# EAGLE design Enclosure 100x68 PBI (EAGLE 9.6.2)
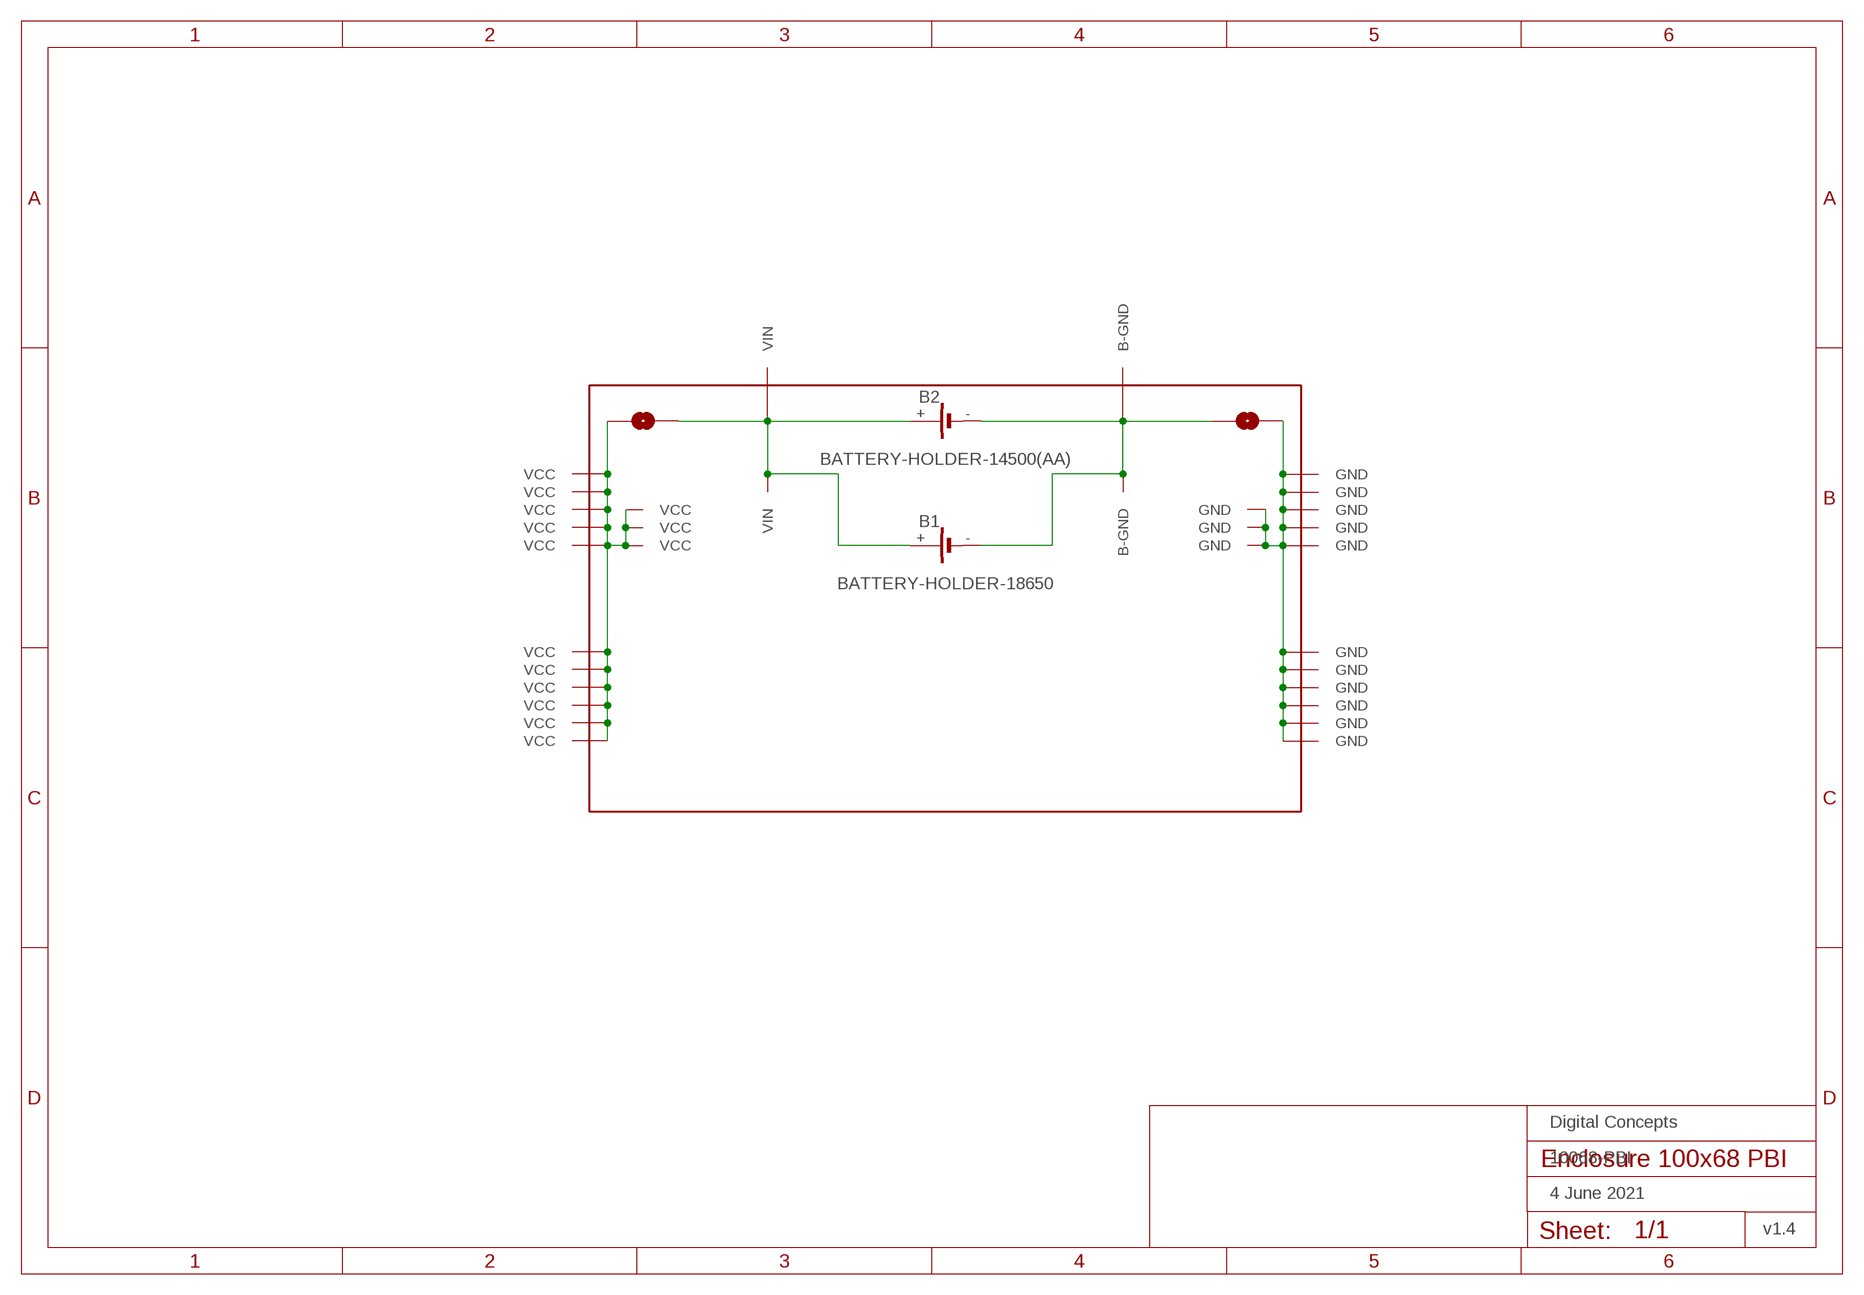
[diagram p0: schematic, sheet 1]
FRAME1 (FRAME-A4L-LOC): DATE: 4 June 2021; OWNER: Digital Concepts; TITLE: 10068-PBI; VERSION: v1.4

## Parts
B1  BATTERY-HOLDER-18650  [BATTERY-18650]
B2  BATTERY-HOLDER-14500(AA)  [BATTERY-14500]
P1  PROTO-34X22-BAT-SJ-MK2  [PROTO-34X22-BAT-SJ-MK2]

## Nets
GND: P1.GND P1.P33-13(GND) P1.P33-14(GND) P1.P33-15(GND) P1.P34-05(GND) P1.P34-06(GND) P1.P34-07(GND) P1.P34-08(GND) P1.P34-09(GND) P1.P34-10(GND) P1.P34-13(GND) P1.P34-14(GND) P1.P34-15(GND) P1.P34-16(GND) P1.P34-17(GND)
N$3: B1.+ B2.+ P1.P02-17(VIN) P1.P05-19(VIN) P1.VIN
N$4: B1.- B2.- P1.B-GND P1.P30-19(B-GND) P1.P33-17(B-GND)
VCC: P1.P01-05(VCC) P1.P01-06(VCC) P1.P01-07(VCC) P1.P01-08(VCC) P1.P01-09(VCC) P1.P01-10(VCC) P1.P01-13(VCC) P1.P01-14(VCC) P1.P01-15(VCC) P1.P01-16(VCC) P1.P01-17(VCC) P1.P02-13(VCC) P1.P02-14(VCC) P1.P02-15(VCC) P1.VCC

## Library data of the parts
B1 = digitalconcepts:BATTERY-HOLDER-18650: 18650 Battery Holder
B2 = digitalconcepts:BATTERY-HOLDER-14500(AA): 14500 (AA) battery holder
P1 = digitalconcepts:PROTO-34X22-BAT-SJ-MK2: 34 x 22 Prototyping board, with spaces for battery connection (GND + Vcc plane) to fit a 100 x 68 enclosure

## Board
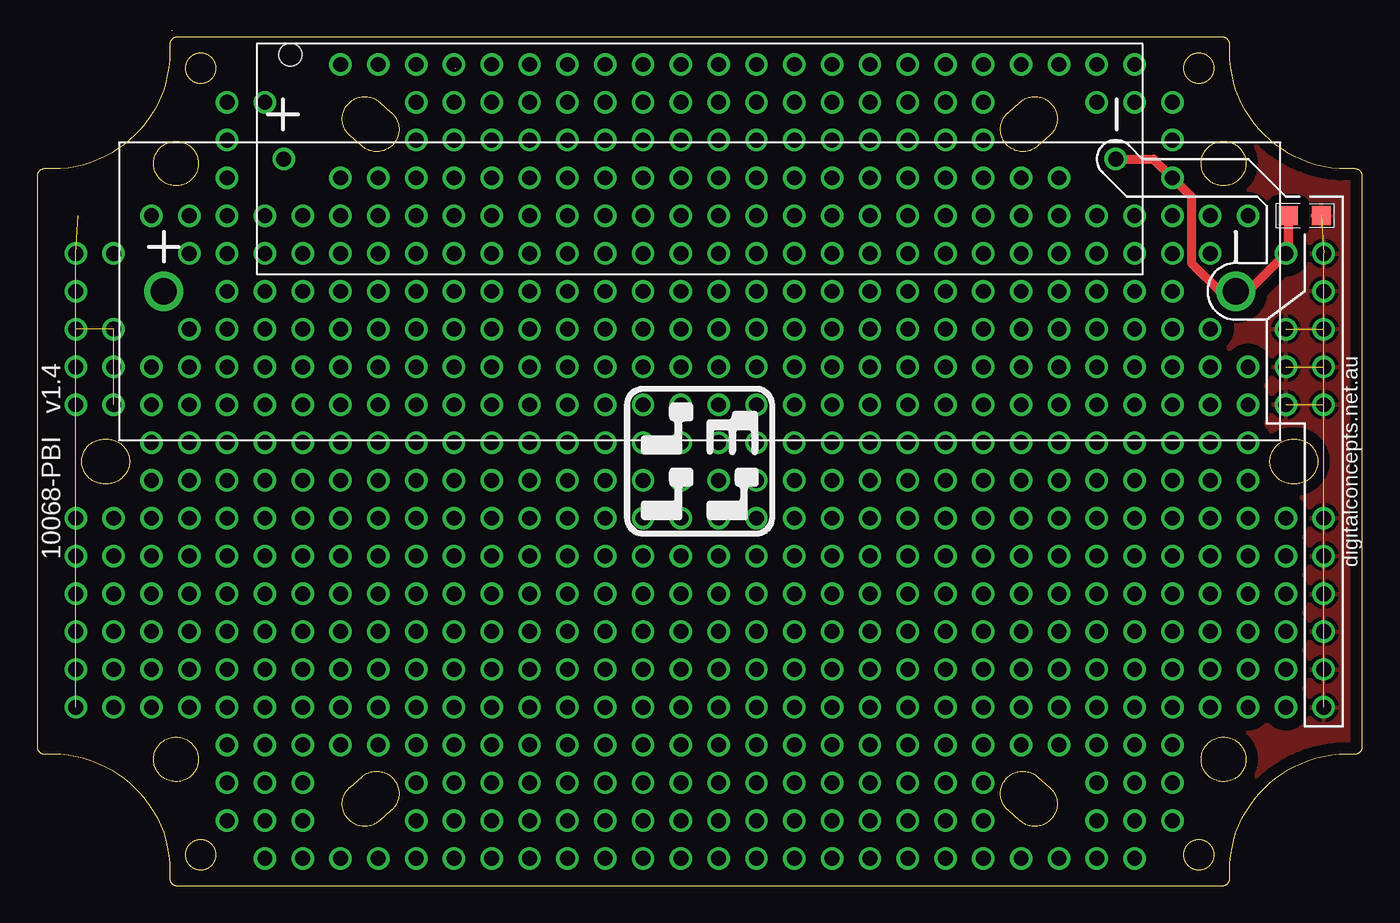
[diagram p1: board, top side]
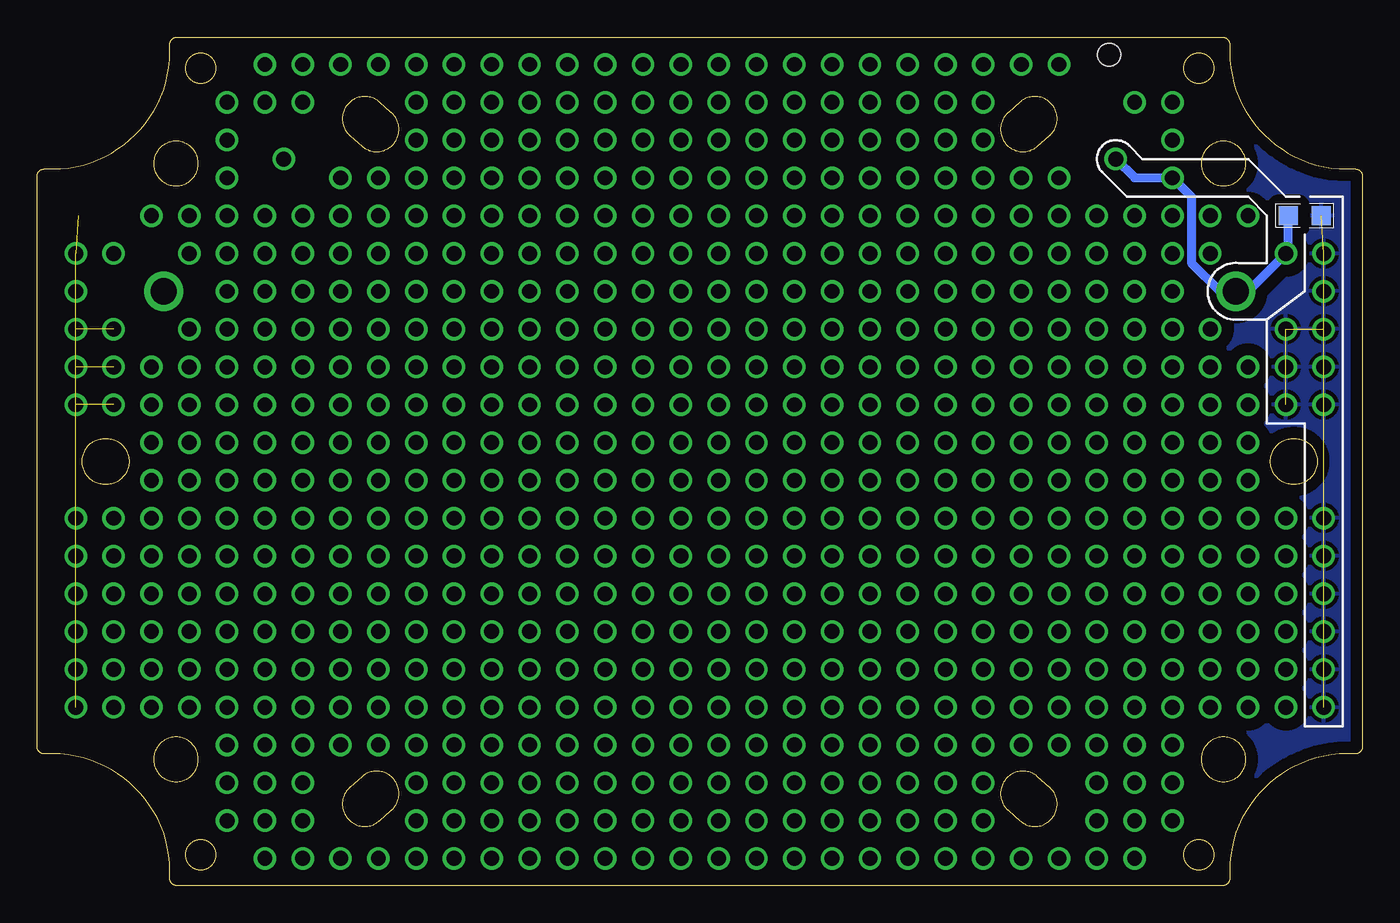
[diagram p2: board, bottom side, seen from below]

Size 89 x 57 mm. Coordinates in mm from the lower left corner, seen from the top.
Outline: 1238 segments
Outline: circle at 10.97,54.92 radius 1.02
Outline: circle at 78.03,54.92 radius 1.02
Outline: circle at 78.03,2.08 radius 1.02
Outline: circle at 10.97,2.08 radius 1.02
Copper layers (1*16): Top 0.035mm / dielectric 1.5mm / Bottom 0.035mm
Design rules "default *": minimum track width 6mil, minimum drill 0.35mm, track to track 6mil, track to pad 6mil, pad to pad 6mil, via to via 6mil, smd to smd 6mil, copper to edge 6mil, drill to drill 6mil, minimum pad ring 10mil, minimum via ring 8mil, stop-mask expansion 4mil, vias tented up to drill 0mil, thermal gap 10mil

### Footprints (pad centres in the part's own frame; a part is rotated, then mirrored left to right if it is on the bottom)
BATTERY-18650 = drill 1.75: + -36,0; - 36,0
BATTERY-14500 = drill 1: + -27.94,0; - 27.94,0 | hole 1.524: -27.5,7
PROTO-34X22-BAT-SJ-MK2 = smd 1.27 x 1.27: B-GND 39.534,16.51; GND 41.746,16.51 | drill 1: P01-05 -41.91,-16.51; P01-06 -41.91,-13.97; P01-07 -41.91,-11.43; P01-08 -41.91,-8.89; P01-09 -41.91,-6.35; P01-10 -41.91,-3.81; P01-13 -41.91,3.81; P01-14 -41.91,6.35; P01-15 -41.91,8.89; P01-16 -41.91,11.43; P01-17 -41.91,13.97; P02-05 -39.37,-16.51; P02-06 -39.37,-13.97; P02-07 -39.37,-11.43; P02-08 -39.37,-8.89; P02-09 -39.37,-6.35; P02-10 -39.37,-3.81; P02-13 -39.37,3.81; P02-14 -39.37,6.35; P02-15 -39.37,8.89; P02-17 -39.37,13.97; P03-05 -36.83,-16.51; P03-06 -36.83,-13.97; P03-07 -36.83,-11.43; P03-08 -36.83,-8.89; P03-09 -36.83,-6.35; P03-10 -36.83,-3.81; P03-11 -36.83,-1.27; P03-12 -36.83,1.27; P03-13 -36.83,3.81; P03-14 -36.83,6.35; P03-18 -36.83,16.51; P04-05 -34.29,-16.51; P04-06 -34.29,-13.97; P04-07 -34.29,-11.43; P04-08 -34.29,-8.89; P04-09 -34.29,-6.35; P04-10 -34.29,-3.81; P04-11 -34.29,-1.27; P04-12 -34.29,1.27; P04-13 -34.29,3.81; P04-14 -34.29,6.35; P04-15 -34.29,8.89; P04-17 -34.29,13.97; P04-18 -34.29,16.51; P05-02 -31.75,-24.13; P05-03 -31.75,-21.59; P05-04 -31.75,-19.05; P05-05 -31.75,-16.51; P05-06 -31.75,-13.97; P05-07 -31.75,-11.43; P05-08 -31.75,-8.89; P05-09 -31.75,-6.35; P05-10 -31.75,-3.81; P05-11 -31.75,-1.27; P05-12 -31.75,1.27; P05-13 -31.75,3.81; P05-14 -31.75,6.35; P05-15 -31.75,8.89; P05-16 -31.75,11.43; P05-17 -31.75,13.97; P05-18 -31.75,16.51; P05-19 -31.75,19.05; P05-20 -31.75,21.59; P05-21 -31.75,24.13; P06-01 -29.21,-26.67; P06-02 -29.21,-24.13; P06-03 -29.21,-21.59; P06-04 -29.21,-19.05; P06-05 -29.21,-16.51; P06-06 -29.21,-13.97; P06-07 -29.21,-11.43; P06-08 -29.21,-8.89; P06-09 -29.21,-6.35; P06-10 -29.21,-3.81; P06-11 -29.21,-1.27; P06-12 -29.21,1.27; P06-13 -29.21,3.81; P06-14 -29.21,6.35; P06-15 -29.21,8.89; P06-16 -29.21,11.43; P06-17 -29.21,13.97; P06-18 -29.21,16.51; P06-21 -29.21,24.13; P07-01 -26.67,-26.67; P07-02 -26.67,-24.13; P07-03 -26.67,-21.59; P07-04 -26.67,-19.05; P07-05 -26.67,-16.51; P07-06 -26.67,-13.97; P07-07 -26.67,-11.43; P07-08 -26.67,-8.89; P07-09 -26.67,-6.35; P07-10 -26.67,-3.81; P07-11 -26.67,-1.27; P07-12 -26.67,1.27; P07-13 -26.67,3.81; P07-14 -26.67,6.35; P07-15 -26.67,8.89; P07-16 -26.67,11.43; P07-17 -26.67,13.97; P07-18 -26.67,16.51; P08-01 -24.13,-26.67; P08-04 -24.13,-19.05; P08-05 -24.13,-16.51; P08-06 -24.13,-13.97; P08-07 -24.13,-11.43; P08-08 -24.13,-8.89; P08-09 -24.13,-6.35; P08-10 -24.13,-3.81; P08-11 -24.13,-1.27; P08-12 -24.13,1.27; P08-13 -24.13,3.81; P08-14 -24.13,6.35; P08-15 -24.13,8.89; P08-16 -24.13,11.43; P08-17 -24.13,13.97; P08-18 -24.13,16.51; P08-19 -24.13,19.05; P08-22 -24.13,26.67; P09-01 -21.59,-26.67; P09-04 -21.59,-19.05; P09-05 -21.59,-16.51; P09-06 -21.59,-13.97; P09-07 -21.59,-11.43; P09-08 -21.59,-8.89; P09-09 -21.59,-6.35; P09-10 -21.59,-3.81; P09-11 -21.59,-1.27; P09-12 -21.59,1.27; P09-13 -21.59,3.81; P09-14 -21.59,6.35; P09-15 -21.59,8.89; P09-16 -21.59,11.43; P09-17 -21.59,13.97; P09-18 -21.59,16.51; P09-19 -21.59,19.05; P09-22 -21.59,26.67; P10-01 -19.05,-26.67; P10-02 -19.05,-24.13; P10-03 -19.05,-21.59; P10-04 -19.05,-19.05; P10-05 -19.05,-16.51; P10-06 -19.05,-13.97; P10-07 -19.05,-11.43; P10-08 -19.05,-8.89; P10-09 -19.05,-6.35; P10-10 -19.05,-3.81; P10-11 -19.05,-1.27; P10-12 -19.05,1.27; P10-13 -19.05,3.81; P10-14 -19.05,6.35; P10-15 -19.05,8.89; P10-16 -19.05,11.43; P10-17 -19.05,13.97; P10-18 -19.05,16.51; P10-19 -19.05,19.05; P10-20 -19.05,21.59; P10-21 -19.05,24.13; P10-22 -19.05,26.67; P11-01 -16.51,-26.67; P11-02 -16.51,-24.13; P11-03 -16.51,-21.59; P11-04 -16.51,-19.05; P11-05 -16.51,-16.51; P11-06 -16.51,-13.97; P11-07 -16.51,-11.43; P11-08 -16.51,-8.89; P11-09 -16.51,-6.35; P11-10 -16.51,-3.81; P11-11 -16.51,-1.27; P11-12 -16.51,1.27; P11-13 -16.51,3.81; P11-14 -16.51,6.35; P11-15 -16.51,8.89; P11-16 -16.51,11.43; P11-17 -16.51,13.97; P11-18 -16.51,16.51; P11-19 -16.51,19.05; P11-20 -16.51,21.59; P11-21 -16.51,24.13; P11-22 -16.51,26.67; P12-01 -13.97,-26.67; P12-02 -13.97,-24.13; P12-03 -13.97,-21.59; P12-04 -13.97,-19.05; P12-05 -13.97,-16.51; P12-06 -13.97,-13.97; P12-07 -13.97,-11.43; P12-08 -13.97,-8.89; P12-09 -13.97,-6.35; P12-10 -13.97,-3.81; P12-11 -13.97,-1.27; P12-12 -13.97,1.27; P12-13 -13.97,3.81; P12-14 -13.97,6.35; P12-15 -13.97,8.89; P12-16 -13.97,11.43; P12-17 -13.97,13.97; P12-18 -13.97,16.51; P12-19 -13.97,19.05; P12-20 -13.97,21.59; P12-21 -13.97,24.13; P12-22 -13.97,26.67; P13-01 -11.43,-26.67; P13-02 -11.43,-24.13; P13-03 -11.43,-21.59; P13-04 -11.43,-19.05; P13-05 -11.43,-16.51; P13-06 -11.43,-13.97; P13-07 -11.43,-11.43; P13-08 -11.43,-8.89; P13-09 -11.43,-6.35; P13-10 -11.43,-3.81; P13-11 -11.43,-1.27; P13-12 -11.43,1.27; P13-13 -11.43,3.81; P13-14 -11.43,6.35; P13-15 -11.43,8.89; P13-16 -11.43,11.43; P13-17 -11.43,13.97; P13-18 -11.43,16.51; P13-19 -11.43,19.05; P13-20 -11.43,21.59; P13-21 -11.43,24.13; P13-22 -11.43,26.67; P14-01 -8.89,-26.67; P14-02 -8.89,-24.13; P14-03 -8.89,-21.59; P14-04 -8.89,-19.05; P14-05 -8.89,-16.51; P14-06 -8.89,-13.97; P14-07 -8.89,-11.43; P14-08 -8.89,-8.89; P14-09 -8.89,-6.35; P14-10 -8.89,-3.81; P14-11 -8.89,-1.27; P14-12 -8.89,1.27; P14-13 -8.89,3.81; P14-14 -8.89,6.35; P14-15 -8.89,8.89; P14-16 -8.89,11.43; P14-17 -8.89,13.97; P14-18 -8.89,16.51; P14-19 -8.89,19.05; P14-20 -8.89,21.59; P14-21 -8.89,24.13; P14-22 -8.89,26.67; P15-01 -6.35,-26.67; P15-02 -6.35,-24.13; P15-03 -6.35,-21.59; P15-04 -6.35,-19.05; P15-05 -6.35,-16.51; P15-06 -6.35,-13.97; P15-07 -6.35,-11.43; P15-08 -6.35,-8.89; P15-09 -6.35,-6.35; P15-10 -6.35,-3.81; P15-11 -6.35,-1.27; P15-12 -6.35,1.27; P15-13 -6.35,3.81; P15-14 -6.35,6.35; P15-15 -6.35,8.89; P15-16 -6.35,11.43; P15-17 -6.35,13.97; P15-18 -6.35,16.51; P15-19 -6.35,19.05; P15-20 -6.35,21.59; P15-21 -6.35,24.13; P15-22 -6.35,26.67; P16-01 -3.81,-26.67; P16-02 -3.81,-24.13; P16-03 -3.81,-21.59; P16-04 -3.81,-19.05; P16-05 -3.81,-16.51; P16-06 -3.81,-13.97; P16-07 -3.81,-11.43; P16-08 -3.81,-8.89; P16-09 -3.81,-6.35; P16-10 -3.81,-3.81; P16-11 -3.81,-1.27; P16-12 -3.81,1.27; P16-13 -3.81,3.81; P16-14 -3.81,6.35; P16-15 -3.81,8.89; P16-16 -3.81,11.43; P16-17 -3.81,13.97; P16-18 -3.81,16.51; P16-19 -3.81,19.05; P16-20 -3.81,21.59; P16-21 -3.81,24.13; P16-22 -3.81,26.67; P17-01 -1.27,-26.67; P17-02 -1.27,-24.13; P17-03 -1.27,-21.59; P17-04 -1.27,-19.05; P17-05 -1.27,-16.51; P17-06 -1.27,-13.97; P17-07 -1.27,-11.43; P17-08 -1.27,-8.89; P17-09 -1.27,-6.35; P17-10 -1.27,-3.81; P17-11 -1.27,-1.27; P17-12 -1.27,1.27; P17-13 -1.27,3.81; P17-14 -1.27,6.35; P17-15 -1.27,8.89; P17-16 -1.27,11.43; P17-17 -1.27,13.97; P17-18 -1.27,16.51; P17-19 -1.27,19.05; P17-20 -1.27,21.59; P17-21 -1.27,24.13; P17-22 -1.27,26.67; P18-01 1.27,-26.67; P18-02 1.27,-24.13; P18-03 1.27,-21.59; P18-04 1.27,-19.05; P18-05 1.27,-16.51; P18-06 1.27,-13.97; P18-07 1.27,-11.43; P18-08 1.27,-8.89; P18-09 1.27,-6.35; P18-10 1.27,-3.81; P18-11 1.27,-1.27; P18-12 1.27,1.27; P18-13 1.27,3.81; P18-14 1.27,6.35; P18-15 1.27,8.89; P18-16 1.27,11.43; P18-17 1.27,13.97; P18-18 1.27,16.51; P18-19 1.27,19.05; P18-20 1.27,21.59; P18-21 1.27,24.13; P18-22 1.27,26.67; P19-01 3.81,-26.67; P19-02 3.81,-24.13; P19-03 3.81,-21.59; P19-04 3.81,-19.05; P19-05 3.81,-16.51; P19-06 3.81,-13.97; P19-07 3.81,-11.43; P19-08 3.81,-8.89; P19-09 3.81,-6.35; P19-10 3.81,-3.81; P19-11 3.81,-1.27; P19-12 3.81,1.27; P19-13 3.81,3.81; P19-14 3.81,6.35; P19-15 3.81,8.89; P19-16 3.81,11.43; P19-17 3.81,13.97; P19-18 3.81,16.51; P19-19 3.81,19.05; P19-20 3.81,21.59; P19-21 3.81,24.13; P19-22 3.81,26.67; P20-01 6.35,-26.67; P20-02 6.35,-24.13; P20-03 6.35,-21.59; P20-04 6.35,-19.05; P20-05 6.35,-16.51; P20-06 6.35,-13.97; P20-07 6.35,-11.43; P20-08 6.35,-8.89; P20-09 6.35,-6.35; P20-10 6.35,-3.81; P20-11 6.35,-1.27; P20-12 6.35,1.27; P20-13 6.35,3.81; P20-14 6.35,6.35; P20-15 6.35,8.89; P20-16 6.35,11.43; P20-17 6.35,13.97; P20-18 6.35,16.51; P20-19 6.35,19.05; P20-20 6.35,21.59; P20-21 6.35,24.13; P20-22 6.35,26.67; P21-01 8.89,-26.67; P21-02 8.89,-24.13; P21-03 8.89,-21.59; P21-04 8.89,-19.05; P21-05 8.89,-16.51; P21-06 8.89,-13.97; P21-07 8.89,-11.43; P21-08 8.89,-8.89; P21-09 8.89,-6.35; P21-10 8.89,-3.81; P21-11 8.89,-1.27; P21-12 8.89,1.27; P21-13 8.89,3.81; P21-14 8.89,6.35; P21-15 8.89,8.89; P21-16 8.89,11.43; P21-17 8.89,13.97; P21-18 8.89,16.51; P21-19 8.89,19.05; P21-20 8.89,21.59; P21-21 8.89,24.13; P21-22 8.89,26.67; P22-01 11.43,-26.67; P22-02 11.43,-24.13; P22-03 11.43,-21.59; P22-04 11.43,-19.05; P22-05 11.43,-16.51; P22-06 11.43,-13.97; P22-07 11.43,-11.43; P22-08 11.43,-8.89; P22-09 11.43,-6.35; P22-10 11.43,-3.81; P22-11 11.43,-1.27; P22-12 11.43,1.27; P22-13 11.43,3.81; P22-14 11.43,6.35; P22-15 11.43,8.89; P22-16 11.43,11.43; P22-17 11.43,13.97; P22-18 11.43,16.51; P22-19 11.43,19.05; P22-20 11.43,21.59; P22-21 11.43,24.13; P22-22 11.43,26.67; P23-01 13.97,-26.67; P23-02 13.97,-24.13; P23-03 13.97,-21.59; P23-04 13.97,-19.05; P23-05 13.97,-16.51; P23-06 13.97,-13.97; P23-07 13.97,-11.43; P23-08 13.97,-8.89; P23-09 13.97,-6.35; P23-10 13.97,-3.81; P23-11 13.97,-1.27; P23-12 13.97,1.27; P23-13 13.97,3.81; P23-14 13.97,6.35; P23-15 13.97,8.89; P23-16 13.97,11.43; P23-17 13.97,13.97; P23-18 13.97,16.51; P23-19 13.97,19.05; P23-20 13.97,21.59; P23-21 13.97,24.13; P23-22 13.97,26.67; P24-01 16.51,-26.67; P24-02 16.51,-24.13; P24-03 16.51,-21.59; P24-04 16.51,-19.05; P24-05 16.51,-16.51; P24-06 16.51,-13.97; P24-07 16.51,-11.43; P24-08 16.51,-8.89; P24-09 16.51,-6.35; P24-10 16.51,-3.81; P24-11 16.51,-1.27; P24-12 16.51,1.27; P24-13 16.51,3.81; P24-14 16.51,6.35; P24-15 16.51,8.89; P24-16 16.51,11.43; P24-17 16.51,13.97; P24-18 16.51,16.51; P24-19 16.51,19.05; P24-20 16.51,21.59; P24-21 16.51,24.13; P24-22 16.51,26.67; P25-01 19.05,-26.67; P25-02 19.05,-24.13; P25-03 19.05,-21.59; P25-04 19.05,-19.05; P25-05 19.05,-16.51; P25-06 19.05,-13.97; P25-07 19.05,-11.43; P25-08 19.05,-8.89; P25-09 19.05,-6.35; P25-10 19.05,-3.81; P25-11 19.05,-1.27; P25-12 19.05,1.27; P25-13 19.05,3.81; P25-14 19.05,6.35; P25-15 19.05,8.89; P25-16 19.05,11.43; P25-17 19.05,13.97; P25-18 19.05,16.51; P25-19 19.05,19.05; P25-20 19.05,21.59; P25-21 19.05,24.13; P25-22 19.05,26.67; P26-01 21.59,-26.67; P26-04 21.59,-19.05; P26-05 21.59,-16.51; P26-06 21.59,-13.97; P26-07 21.59,-11.43; P26-08 21.59,-8.89; P26-09 21.59,-6.35; P26-10 21.59,-3.81; P26-11 21.59,-1.27; P26-12 21.59,1.27; P26-13 21.59,3.81; P26-14 21.59,6.35; P26-15 21.59,8.89; P26-16 21.59,11.43; P26-17 21.59,13.97; P26-18 21.59,16.51; P26-19 21.59,19.05; P26-22 21.59,26.67; P27-01 24.13,-26.67; P27-04 24.13,-19.05; P27-05 24.13,-16.51; P27-06 24.13,-13.97; P27-07 24.13,-11.43; P27-08 24.13,-8.89; P27-09 24.13,-6.35; P27-10 24.13,-3.81; P27-11 24.13,-1.27; P27-12 24.13,1.27; P27-13 24.13,3.81; P27-14 24.13,6.35; P27-15 24.13,8.89; P27-16 24.13,11.43; P27-17 24.13,13.97; P27-18 24.13,16.51; P27-19 24.13,19.05; P27-22 24.13,26.67; P28-01 26.67,-26.67; P28-02 26.67,-24.13; P28-03 26.67,-21.59; P28-04 26.67,-19.05; P28-05 26.67,-16.51; P28-06 26.67,-13.97; P28-07 26.67,-11.43; P28-08 26.67,-8.89; P28-09 26.67,-6.35; P28-10 26.67,-3.81; P28-11 26.67,-1.27; P28-12 26.67,1.27; P28-13 26.67,3.81; P28-14 26.67,6.35; P28-15 26.67,8.89; P28-16 26.67,11.43; P28-17 26.67,13.97; P28-18 26.67,16.51; P28-21 26.67,24.13; P28-22 26.67,26.67; P29-01 29.21,-26.67; P29-02 29.21,-24.13; P29-03 29.21,-21.59; P29-04 29.21,-19.05; P29-05 29.21,-16.51; P29-06 29.21,-13.97; P29-07 29.21,-11.43; P29-08 29.21,-8.89; P29-09 29.21,-6.35; P29-10 29.21,-3.81; P29-11 29.21,-1.27; P29-12 29.21,1.27; P29-13 29.21,3.81; P29-14 29.21,6.35; P29-15 29.21,8.89; P29-16 29.21,11.43; P29-17 29.21,13.97; P29-18 29.21,16.51; P29-21 29.21,24.13; P29-22 29.21,26.67; P30-02 31.75,-24.13; P30-03 31.75,-21.59; P30-04 31.75,-19.05; P30-05 31.75,-16.51; P30-06 31.75,-13.97; P30-07 31.75,-11.43; P30-08 31.75,-8.89; P30-09 31.75,-6.35; P30-10 31.75,-3.81; P30-11 31.75,-1.27; P30-12 31.75,1.27; P30-13 31.75,3.81; P30-14 31.75,6.35; P30-15 31.75,8.89; P30-16 31.75,11.43; P30-17 31.75,13.97; P30-18 31.75,16.51; P30-19 31.75,19.05; P30-20 31.75,21.59; P30-21 31.75,24.13; P31-05 34.29,-16.51; P31-06 34.29,-13.97; P31-07 34.29,-11.43; P31-08 34.29,-8.89; P31-09 34.29,-6.35; P31-10 34.29,-3.81; P31-11 34.29,-1.27; P31-12 34.29,1.27; P31-13 34.29,3.81; P31-14 34.29,6.35; P31-15 34.29,8.89; P31-17 34.29,13.97; P31-18 34.29,16.51; P32-05 36.83,-16.51; P32-06 36.83,-13.97; P32-07 36.83,-11.43; P32-08 36.83,-8.89; P32-09 36.83,-6.35; P32-10 36.83,-3.81; P32-11 36.83,-1.27; P32-12 36.83,1.27; P32-13 36.83,3.81; P32-14 36.83,6.35; P32-18 36.83,16.51; P33-05 39.37,-16.51; P33-06 39.37,-13.97; P33-07 39.37,-11.43; P33-08 39.37,-8.89; P33-09 39.37,-6.35; P33-10 39.37,-3.81; P33-13 39.37,3.81; P33-14 39.37,6.35; P33-15 39.37,8.89; P33-17 39.37,13.97; P34-05 41.91,-16.51; P34-06 41.91,-13.97; P34-07 41.91,-11.43; P34-08 41.91,-8.89; P34-09 41.91,-6.35; P34-10 41.91,-3.81; P34-13 41.91,3.81; P34-14 41.91,6.35; P34-15 41.91,8.89; P34-16 41.91,11.43; P34-17 41.91,13.97 | smd 1.27 x 1.27 bottom: VCC -41.746,16.51; VIN -39.534,16.51

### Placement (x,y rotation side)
B1  44.5,39.93 0 top
B2  44.5,48.82 0 top
P1  44.5,28.5 0 top

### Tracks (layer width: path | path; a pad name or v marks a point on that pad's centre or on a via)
GND  (14 unrouted)
  pour Top (isolate 0.813): -1.98,58.98 -1.98,-1.98 91.11,-1.98 91.11,58.98
N$3
  Bottom 0.61: B2.+ 15.29,47.55 P1.P05-19 11.48,46.28 11.48,41.83 9.57,39.93 B1.+ 7.67,39.93 P1.P02-17 4.97,42.63 P1.VIN
N$4
  Top 0.61: B2.- 74.98,48.82 P1.P30-19 77.52,46.28 77.52,41.83 79.42,39.93 B1.- 81.33,39.93 P1.P33-17 84.03,42.63 P1.B-GND
VCC  (14 unrouted)
  pour Bottom (isolate 0.813): -0.71,57.71 -0.71,-0.71 89.84,-0.71 89.84,57.71

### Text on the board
tPlace: 10068-PBI v1.4 | digitalconcepts.net.au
